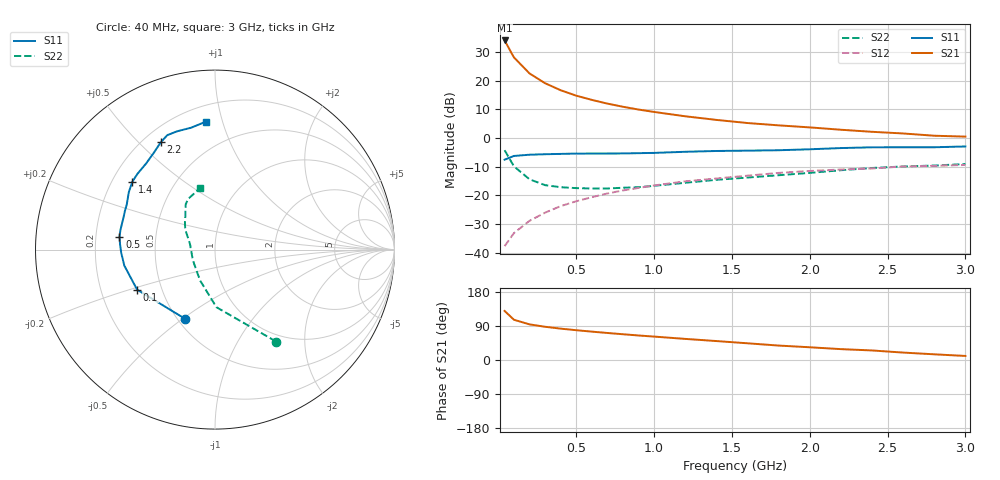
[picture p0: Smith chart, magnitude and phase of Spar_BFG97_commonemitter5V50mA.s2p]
! Filename:  BFG97C.S2P  Version:  2.0
! NXP part #: BFG97  Date: Jul 1990
! Bias condition: Vce=5V, Ic=50mA
#  MHz  S  MA  R  50
! Freq  S11  S21  S12  S22  !GUM [dB]
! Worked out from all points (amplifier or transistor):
!   21 points, 40 MHz to 3 GHz, reference 50 ohm
!   highest |S21| = 34.1 dB at 40 MHz (marker M1)
!   |S21| within 3 dB of that: start of sweep to 70.42 MHz
!   unconditionally stable (mu >= 1): 240.7 MHz to 2.981 GHz
!   at 300 MHz: K = 1.04, MAG = 21.4 dB, |S12| = -26.0 dB
!   at 1 GHz: K = 1.09, MAG = 11.0 dB, |S12| = -16.5 dB
!   at 3 GHz: K = 1.00, MSG = 4.9 dB, |S12| = -9.4 dB
!   S11 on the Smith chart (normalised r, x): 40 MHz: 0.55, -0.51; 100 MHz: 0.36, -0.21; 500 MHz: 0.30, +0.06; 1.4 GHz: 0.28, +0.33; 2.2 GHz: 0.27, +0.58; 3 GHz: 0.30, +0.88
40  0.42 -113.4  50.61 129.5  0.013 63.8  0.615 -56.4
100  0.488 -152.8  25.61 106.2  0.022 63.3  0.321 -88.6
200  0.513 -170.0  13.45 94.0  0.036 67.7  0.191 -115.8
300  0.523 -178.1  9.075 87.7  0.05 69.9  0.151 -134.8
400  0.53 176.7  6.846 82.8  0.065 71.0  0.139 -148.6
500  0.537 172.3  5.506 78.6  0.079 70.3  0.134 -159.6
600  0.538 168.4  4.647 74.9  0.093 70.0  0.132 -167.7
700  0.538 164.7  4 71.3  0.108 69.3  0.132 -175.2
800  0.54 160.8  3.525 68.0  0.122 67.6  0.136 177.7
900  0.546 156.9  3.151 64.7  0.135 66.9  0.139 171.0
1000  0.552 153.0  2.862 61.8  0.149 65.6  0.147 164.7
1200  0.577 146.3  2.404 55.7  0.176 62.5  0.166 155.6
1400  0.596 140.6  2.079 50.0  0.197 59.6  0.187 149.2
1600  0.604 135.7  1.833 44.1  0.221 57.5  0.205 144.1
1800  0.614 128.8  1.669 38.1  0.247 52.8  0.225 138.1
2000  0.638 122.3  1.538 33.6  0.267 50.7  0.247 132.0
2200  0.67 116.8  1.4 28.7  0.283 47.3  0.275 126.8
2400  0.691 112.6  1.288 25.2  0.295 46.2  0.301 122.8
2600  0.692 107.6  1.205 19.6  0.32 42.2  0.32 117.7
2800  0.692 101.0  1.1 15.0  0.328 37.3  0.332 111.0
3000  0.715 94.1  1.062 10.7  0.34 35.6  0.353 104.0
